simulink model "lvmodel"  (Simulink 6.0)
settings: Solver=ode45  StartTime=0.0  StopTime=200.0  RelTol=1e-3

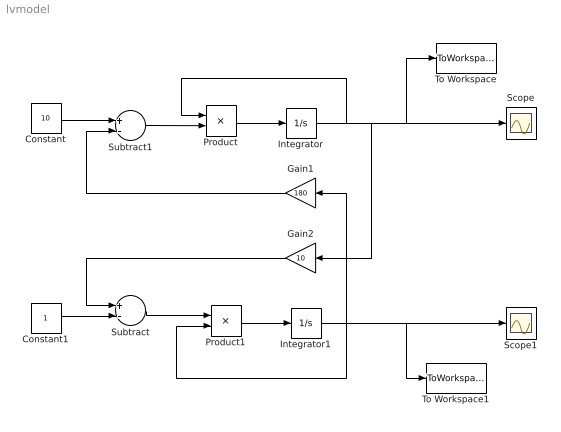
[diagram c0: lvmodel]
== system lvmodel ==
  Constant : Constant  Value=10
  Constant1 : Constant
  Gain1 : Gain  Orientation=left  Gain=180
  Gain2 : Gain  Orientation=left  Gain=10
  Integrator : Integrator  InitialCondition=0.8
  Integrator1 : Integrator  InitialCondition=0.8
  Product : Product
  Product1 : Product
  Scope : Scope
  Scope1 : Scope
  Subtract : Sum  Inputs=+-  OutScaling=2^-10
  Subtract1 : Sum  Inputs=+-  OutScaling=2^-10
  To Workspace : ToWorkspace  VariableName=prey  SampleTime=-1  SaveFormat=Array
  To Workspace1 : ToWorkspace  VariableName=predator  SampleTime=-1  SaveFormat=Array
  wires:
  Product1/1 -> Integrator1/1
  Product/1 -> Integrator/1
  Integrator1/1 -> Gain1/1, Product1/2, To Workspace1/1, Scope1/1
  Integrator/1 -> Gain2/1, To Workspace/1, Scope/1, Product/1
  Gain1/1 -> Subtract1/2
  Gain2/1 -> Subtract/1
  Subtract/1 -> Product1/1
  Constant/1 -> Subtract1/1
  Constant1/1 -> Subtract/2
  Subtract1/1 -> Product/2
